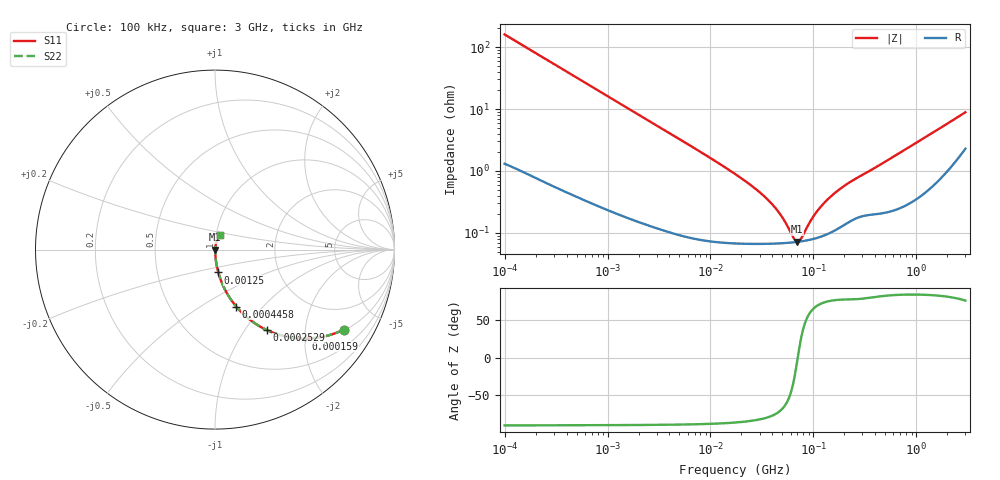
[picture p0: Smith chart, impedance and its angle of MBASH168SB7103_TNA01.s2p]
! MBASH168SB7103_TNA01  S-PARAMETER MODEL  ( Standard Model )
! Model Generated by TAIYO YUDEN Corporation (http://www.ty-top.com)
! Version 1.0
! TAIYO YUDEN Control No. 220601
! Copyright(c) 2013 TAIYO YUDEN CO.,LTD. All Rights Reserved.
! Product Description (link to TY-COMPAS)
! https://ds.yuden.co.jp/TYCOMPAS/or/detail?pn=MBASH168SB7103KTNA01&u=M
! Products Name : Multilayer Ceramic Capacitors
! Characteristics :
!  Capacitance : 0.01 [uF] , Rated Voltage : 100 [V] , TCC : X7R
!  Case Size : 1.6 x 0.8 / 0.063 x 0.031 [mm/inch] , Thickness : 0.8 / 0.031 [mm/inch]
!  (Conditions: Temperature = 25 [degC] , DC Bias Voltage = 0 [V])
! External Node Assignments :
!  1  o---| |---o  2
! GND o---------o GND
! Frequency Range : 100kHz  -  3GHz  [ 401 STEP ]
# MHZ S RI R 50
! Freq[MHz].  S11 Real  S11 Imag  S21 Real  S21 Imag  S12 Real  S12 Imag  S22 Real  S22 Imag
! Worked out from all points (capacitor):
!   401 points, 100 kHz to 3 GHz, reference 50 ohm
!   read as one part in series: C = 9.95 nF near 105.3 kHz
!   lowest |Z| = 71.8 mohm at 69.66 MHz (marker M1)
!   series resonance near 70.53 MHz, so ESL is about 510 pH
!   S11 on the Smith chart (normalised r, x): 100 kHz: 1.03, -3.19; 159 kHz: 1.02, -2.01; 252.9 kHz: 1.01, -1.27; 445.8 kHz: 1.01, -0.72; 1.25 MHz: 1.00, -0.26; 3 GHz: 1.05, +0.17
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0.1  0.7168 -0.4465  0.2832 0.4465  0.2832 0.4465  0.7168 -0.4465
0.159027  0.5035 -0.4954  0.4965 0.4954  0.4965 0.4954  0.5035 -0.4954
0.252895  0.2893 -0.4484  0.7107 0.4484  0.7107 0.4484  0.2893 -0.4484
0.335785  0.1893 -0.3864  0.8107 0.3864  0.8107 0.3864  0.1893 -0.3864
0.445844  0.1184 -0.3173  0.8816 0.3173  0.8816 0.3173  0.1184 -0.3173
0.562235  0.0789 -0.2635  0.9211 0.2635  0.9211 0.2635  0.0789 -0.2635
1.249956  0.0185 -0.1272  0.9815 0.1272  0.9815 0.1272  0.0185 -0.1272
3.161081  0.0038 -0.0514  0.9962 0.0514  0.9962 0.0514  0.0038 -0.0514
17.7727  0.000749 -0.00867  0.9993 0.00867  0.9993 0.00867  0.000749 -0.00867
28.26337  0.000687 -0.00489  0.9993 0.00489  0.9993 0.00489  0.000687 -0.00489
39.51212  0.000677 -0.00286  0.9993 0.00286  0.9993 0.00286  0.000677 -0.00286
49.82709  0.000683 -0.00165  0.9993 0.00165  0.9993 0.00165  0.000683 -0.00165
64.47533  0.000705 -0.000419  0.9993 0.000419  0.9993 0.000419  0.000705 -0.000419
69.65816  0.000715 -5.79e-05  0.9993 5.79e-05  0.9993 5.79e-05  0.000715 -5.79e-05
73.34282  0.000723 0.000183  0.9993 -0.000183  0.9993 -0.000183  0.000723 0.000183
77.22239  0.000733 0.000423  0.9993 -0.000423  0.9993 -0.000423  0.000733 0.000423
97.38194  0.000792 0.00153  0.9992 -0.00153  0.9992 -0.00153  0.000792 0.00153
126.0104  0.00091 0.00285  0.9991 -0.00285  0.9991 -0.00285  0.00091 0.00285
176.1623  0.00121 0.00478  0.9988 -0.00478  0.9988 -0.00478  0.00121 0.00478
233.9019  0.00161 0.00662  0.9984 -0.00662  0.9984 -0.00662  0.00161 0.00662
547.5153  0.00242 0.0153  0.9976 -0.0153  0.9976 -0.0153  0.00242 0.0153
3000  0.0292 0.0812  0.9708 -0.0812  0.9708 -0.0812  0.0292 0.0812
